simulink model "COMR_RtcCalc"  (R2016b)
settings: Solver=FixedStepDiscrete  StartTime=0.0  StopTime=10.0  FixedStep=0.1  RelTol=1e-3  EnableMultiTasking=on
undefined symbols (not defined in the file or in its folder): bin2dec, COMR_tiT37FVld_C, COMR_tiTmt2_C
libraries: simulink x3

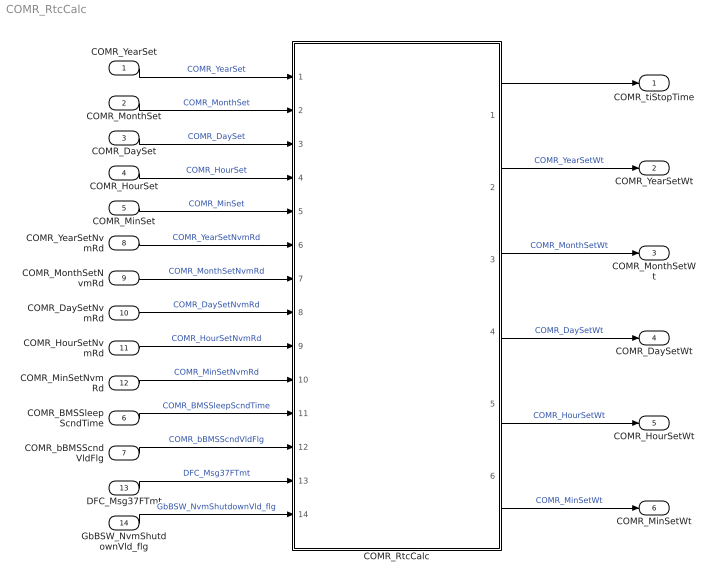
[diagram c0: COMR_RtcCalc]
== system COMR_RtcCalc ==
  COMR_YearSet : Inport
  COMR_MonthSet : Inport  Port=2
  COMR_DaySet : Inport  Port=3
  COMR_HourSet : Inport  Port=4
  COMR_MinSet : Inport  Port=5
  COMR_BMSSleepScndTime : Inport  Port=6
  COMR_bBMSScndVldFlg : Inport  Port=7
  COMR_YearSetNvmRd : Inport  Port=8
  COMR_MonthSetNvmRd : Inport  Port=9
  COMR_DaySetNvmRd : Inport  Port=10
  COMR_HourSetNvmRd : Inport  Port=11
  COMR_MinSetNvmRd : Inport  Port=12
  DFC_Msg37FTmt : Inport  Port=13
  GbBSW_NvmShutdownVld_flg : Inport  Port=14
  COMR_RtcCalc : Subsystem
  COMR_tiStopTime : Outport
  COMR_YearSetWt : Outport  Port=2  InitialOutput=[0]
  COMR_MonthSetWt : Outport  Port=3  InitialOutput=[0]
  COMR_DaySetWt : Outport  Port=4  InitialOutput=[0]
  COMR_HourSetWt : Outport  Port=5  InitialOutput=[0]
  COMR_MinSetWt : Outport  Port=6  InitialOutput=[0]
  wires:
  COMR_YearSet/1 -> COMR_RtcCalc/1(COMR_YearSet)  "COMR_YearSet"
  COMR_MonthSet/1 -> COMR_RtcCalc/2(COMR_MonthSet)  "COMR_MonthSet"
  COMR_DaySet/1 -> COMR_RtcCalc/3(COMR_DaySet)  "COMR_DaySet"
  COMR_HourSet/1 -> COMR_RtcCalc/4(COMR_HourSet)  "COMR_HourSet"
  COMR_RtcCalc/1(COMR_tiStopTime) -> COMR_tiStopTime/1
  COMR_BMSSleepScndTime/1 -> COMR_RtcCalc/11(COMR_BMSSleepScndTime)  "COMR_BMSSleepScndTime"
  COMR_bBMSScndVldFlg/1 -> COMR_RtcCalc/12(COMR_bBMSScndVldFlg)  "COMR_bBMSScndVldFlg"
  COMR_MinSet/1 -> COMR_RtcCalc/5(COMR_MinSet)  "COMR_MinSet"
  COMR_YearSetNvmRd/1 -> COMR_RtcCalc/6(COMR_YearSetNvmRd)  "COMR_YearSetNvmRd"
  COMR_MonthSetNvmRd/1 -> COMR_RtcCalc/7(COMR_MonthSetNvmRd)  "COMR_MonthSetNvmRd"
  COMR_DaySetNvmRd/1 -> COMR_RtcCalc/8(COMR_DaySetNvmRd)  "COMR_DaySetNvmRd"
  COMR_HourSetNvmRd/1 -> COMR_RtcCalc/9(COMR_HourSetNvmRd)  "COMR_HourSetNvmRd"
  COMR_MinSetNvmRd/1 -> COMR_RtcCalc/10(COMR_MinSetNvmRd)  "COMR_MinSetNvmRd"
  COMR_RtcCalc/2(COMR_YearSetWt) -> COMR_YearSetWt/1  "COMR_YearSetWt"
  COMR_RtcCalc/3(COMR_MonthSetWt) -> COMR_MonthSetWt/1  "COMR_MonthSetWt"
  COMR_RtcCalc/4(COMR_DaySetWt) -> COMR_DaySetWt/1  "COMR_DaySetWt"
  COMR_RtcCalc/5(COMR_HourSetWt) -> COMR_HourSetWt/1  "COMR_HourSetWt"
  COMR_RtcCalc/6(COMR_MinSetWt) -> COMR_MinSetWt/1  "COMR_MinSetWt"
  DFC_Msg37FTmt/1 -> COMR_RtcCalc/13(DFC_Msg37FTmt)  "DFC_Msg37FTmt"
  GbBSW_NvmShutdownVld_flg/1 -> COMR_RtcCalc/14(GbBSW_NvmShutdownVld_flg)  "GbBSW_NvmShutdownVld_flg"

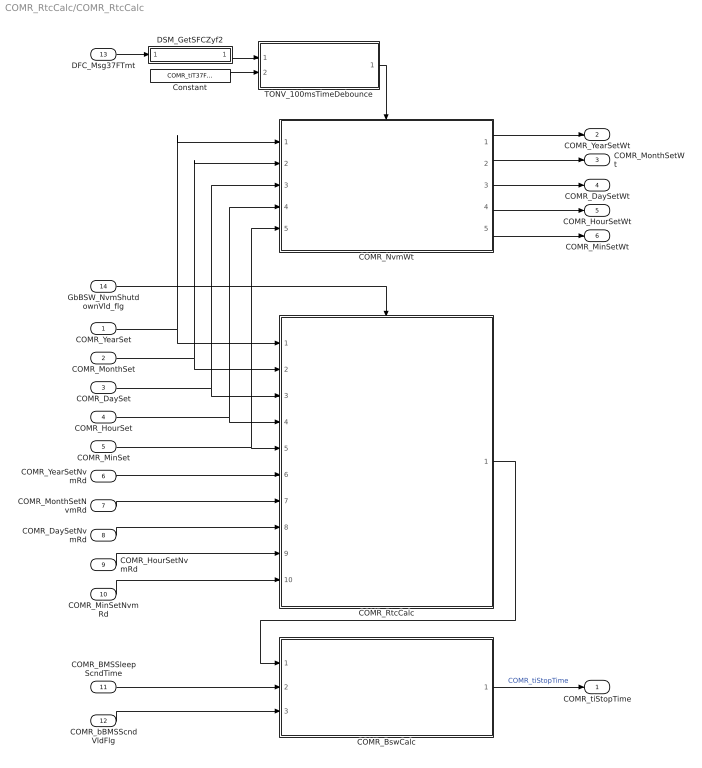
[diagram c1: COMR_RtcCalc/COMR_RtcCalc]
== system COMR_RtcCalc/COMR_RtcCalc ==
  COMR_YearSet : Inport
  COMR_MonthSet : Inport  Port=2
  COMR_DaySet : Inport  Port=3
  COMR_HourSet : Inport  Port=4
  COMR_MinSet : Inport  Port=5
  COMR_YearSetNvmRd : Inport  Port=6
  COMR_MonthSetNvmRd : Inport  Port=7
  COMR_DaySetNvmRd : Inport  Port=8
  COMR_HourSetNvmRd : Inport  Port=9
  COMR_MinSetNvmRd : Inport  Port=10
  COMR_BMSSleepScndTime : Inport  Port=11
  COMR_bBMSScndVldFlg : Inport  Port=12
  DFC_Msg37FTmt : Inport  Port=13
  GbBSW_NvmShutdownVld_flg : Inport  Port=14
  COMR_BswCalc : Subsystem
  COMR_NvmWt : Subsystem
  COMR_RtcCalc : Subsystem
  Constant : Constant  Value=COMR_tiT37FVld_C
  DSM_GetSFCZyf2 : Subsystem  TreatAsAtomicUnit=on  RTWFcnName=TONV_10msTimeDebounce  RTWFileName=SrvLib
  TONV_100msTimeDebounce : Subsystem  TreatAsAtomicUnit=on  RTWFcnName=TONV_100msTimeDebounce  RTWFileName=SrvLib
  COMR_tiStopTime : Outport
  COMR_YearSetWt : Outport  Port=2  InitialOutput=[0]
  COMR_MonthSetWt : Outport  Port=3  InitialOutput=[0]
  COMR_DaySetWt : Outport  Port=4  InitialOutput=[0]
  COMR_HourSetWt : Outport  Port=5  InitialOutput=[0]
  COMR_MinSetWt : Outport  Port=6  InitialOutput=[0]
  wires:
  COMR_YearSetNvmRd/1 -> COMR_RtcCalc/6(COMR_YearSetNvmRd)
  COMR_MonthSetNvmRd/1 -> COMR_RtcCalc/7(COMR_MonthSetNvmRd)
  COMR_MonthSet/1 -> COMR_NvmWt/2(In2), COMR_RtcCalc/2(COMR_MonthSet)
  COMR_DaySet/1 -> COMR_NvmWt/3(In3), COMR_RtcCalc/3(COMR_DaySet)
  COMR_HourSet/1 -> COMR_NvmWt/4(In4), COMR_RtcCalc/4(COMR_HourSet)
  COMR_MinSetNvmRd/1 -> COMR_RtcCalc/10(COMR_MinSetNvmRd)
  COMR_BswCalc/1(COMR_tiStopTime) -> COMR_tiStopTime/1  "COMR_tiStopTime"
  COMR_DaySetNvmRd/1 -> COMR_RtcCalc/8(COMR_DaySetNvmRd)
  COMR_HourSetNvmRd/1 -> COMR_RtcCalc/9(COMR_HourSetNvmRd)
  COMR_YearSet/1 -> COMR_NvmWt/1(In1), COMR_RtcCalc/1(COMR_YearSet)
  COMR_BMSSleepScndTime/1 -> COMR_BswCalc/2(COMR_BMSSleepScndTime)
  COMR_bBMSScndVldFlg/1 -> COMR_BswCalc/3(COMR_bBMSScndVldFlg)
  COMR_RtcCalc/1(COMR_tiStopRtcTime) -> COMR_BswCalc/1(COMR_tiStopRtcTime)
  COMR_MinSet/1 -> COMR_NvmWt/5(In5), COMR_RtcCalc/5(COMR_MinSet)
  COMR_NvmWt/1(COMR_YearSetWt) -> COMR_YearSetWt/1
  COMR_NvmWt/2(COMR_MonthSetWt) -> COMR_MonthSetWt/1
  COMR_NvmWt/3(COMR_DaySetWt) -> COMR_DaySetWt/1
  COMR_NvmWt/4(COMR_HourSetWt) -> COMR_HourSetWt/1
  COMR_NvmWt/5(COMR_MinSetWt) -> COMR_MinSetWt/1
  Constant/1 -> TONV_100msTimeDebounce/2(T)
  TONV_100msTimeDebounce/1(y) -> COMR_NvmWt/Enable
  DSM_GetSFCZyf2/1(y) -> TONV_100msTimeDebounce/1(u)
  DFC_Msg37FTmt/1 -> DSM_GetSFCZyf2/1(DFC)
  GbBSW_NvmShutdownVld_flg/1 -> COMR_RtcCalc/Enable

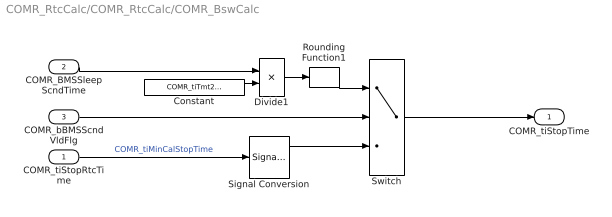
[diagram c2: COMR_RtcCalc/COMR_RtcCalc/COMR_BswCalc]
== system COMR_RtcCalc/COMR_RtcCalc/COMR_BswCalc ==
  COMR_tiStopRtcTime : Inport
  COMR_BMSSleepScndTime : Inport  Port=2
  COMR_bBMSScndVldFlg : Inport  Port=3
  Constant : Constant  Value=COMR_tiTmt2_C  OutDataTypeStr=single
  Divide1 : Product  Inputs=*/
  Rounding Function1 : Rounding
  Signal Conversion : SignalConversion  OverrideOpt=off
  Switch : Switch  Criteria=u2 ~= 0
  COMR_tiStopTime : Outport
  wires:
  COMR_bBMSScndVldFlg/1 -> Switch/2
  COMR_BMSSleepScndTime/1 -> Divide1/1
  COMR_tiStopRtcTime/1 -> Signal Conversion/1  "COMR_tiMinCalStopTime"
  Switch/1 -> COMR_tiStopTime/1
  Rounding Function1/1 -> Switch/1
  Constant/1 -> Divide1/2
  Divide1/1 -> Rounding Function1/1
  Signal Conversion/1 -> Switch/3

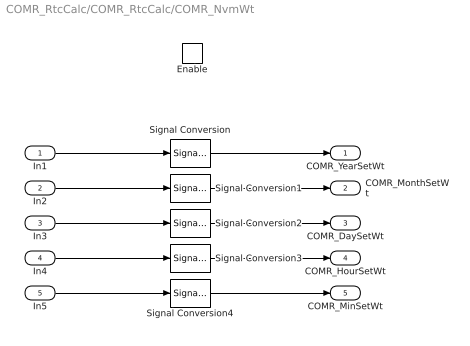
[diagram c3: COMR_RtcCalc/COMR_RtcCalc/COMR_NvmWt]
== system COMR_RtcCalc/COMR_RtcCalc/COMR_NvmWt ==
  In1 : Inport
  In2 : Inport  Port=2
  In3 : Inport  Port=3
  In4 : Inport  Port=4
  In5 : Inport  Port=5
  Enable : EnablePort  StatesWhenEnabling=reset
  Signal Conversion{,1..4} (5 alike) : SignalConversion  OverrideOpt=off
  COMR_YearSetWt : Outport  InitialOutput=[0]
  COMR_MonthSetWt : Outport  Port=2  InitialOutput=[0]
  COMR_DaySetWt : Outport  Port=3  InitialOutput=[0]
  COMR_HourSetWt : Outport  Port=4  InitialOutput=[0]
  COMR_MinSetWt : Outport  Port=5  InitialOutput=[0]
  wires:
  In3/1 -> Signal Conversion2/1
  Signal Conversion/1 -> COMR_YearSetWt/1
  Signal Conversion1/1 -> COMR_MonthSetWt/1
  In1/1 -> Signal Conversion/1
  Signal Conversion2/1 -> COMR_DaySetWt/1
  Signal Conversion3/1 -> COMR_HourSetWt/1
  Signal Conversion4/1 -> COMR_MinSetWt/1
  In4/1 -> Signal Conversion3/1
  In2/1 -> Signal Conversion1/1
  In5/1 -> Signal Conversion4/1

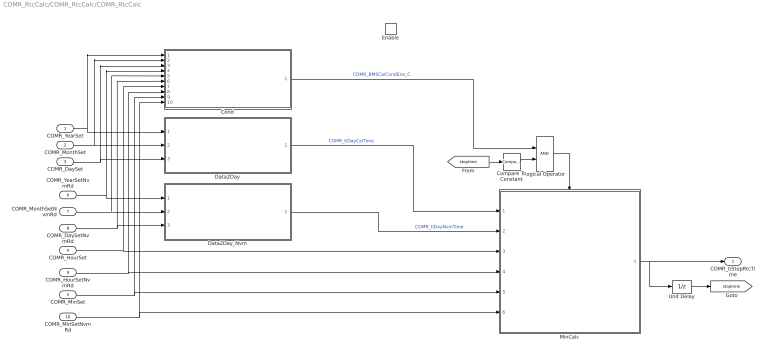
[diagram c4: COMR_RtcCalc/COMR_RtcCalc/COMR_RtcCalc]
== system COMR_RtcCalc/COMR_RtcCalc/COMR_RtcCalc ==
  COMR_YearSet : Inport
  COMR_MonthSet : Inport  Port=2
  COMR_DaySet : Inport  Port=3
  COMR_HourSet : Inport  Port=4
  COMR_MinSet : Inport  Port=5
  COMR_YearSetNvmRd : Inport  Port=6
  COMR_MonthSetNvmRd : Inport  Port=7
  COMR_DaySetNvmRd : Inport  Port=8
  COMR_HourSetNvmRd : Inport  Port=9
  COMR_MinSetNvmRd : Inport  Port=10
  Enable : EnablePort  StatesWhenEnabling=reset
  Compare To Constant : simulink/Logic and Bit Operations/Compare To Constant  relop=<=  const=0  OutDataTypeStr=boolean
  Cond : Subsystem
  Data2Day : Subsystem
  Data2Day_Nvm : Subsystem
  Logical Operator : Logic  AllPortsSameDT=off  OutDataTypeStr=boolean
  MinCalc : Subsystem
  Unit Delay : UnitDelay  SampleTime=-1
  COMR_tiStopRtcTime : Outport  InitialOutput=[0]
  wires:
  MinCalc/1(COMR_tiStopTime) -> Unit Delay/1, COMR_tiStopRtcTime/1
  COMR_YearSet/1 -> Cond/1(COMR_BMSYear), Data2Day/1(BSER_tiYearSet)
  COMR_DaySet/1 -> Cond/3(COMR_BMSDay), Data2Day/3(BSER_tiDaySet)
  COMR_MonthSet/1 -> Cond/2(COMR_BMSMonth), Data2Day/2(BSER_tiMonthSet)
  COMR_YearSetNvmRd/1 -> Cond/4(COMR_BMSYear_nvm), Data2Day_Nvm/1(COMR_BMSYear_nvm)
  COMR_MonthSetNvmRd/1 -> Cond/5(COMR_BMSMonth_nvm), Data2Day_Nvm/2(COMR_BMSMonth_nvm)
  COMR_DaySetNvmRd/1 -> Cond/6(COMR_BMSDay_nvm), Data2Day_Nvm/3(COMR_BMSDay_nvm)
  COMR_HourSet/1 -> Cond/7(COMR_BMSHour), MinCalc/3(COMR_BMSHour)
  COMR_HourSetNvmRd/1 -> Cond/8(COMR_BMSHour_nvm), MinCalc/4(COMR_BMSHour_nvm)
  COMR_MinSetNvmRd/1 -> Cond/10(COMR_BMSMinute_nvm), MinCalc/6(COMR_BMSMinute_nvm)
  COMR_MinSet/1 -> Cond/9(COMR_BMSMinute), MinCalc/5(COMR_BMSMinute)
  Data2Day/1(BSER_tiDay) -> MinCalc/1(BSER_tiDay)  "COMR_tiDayCalTime"
  Data2Day_Nvm/1(BSER_tiDay_nvm) -> MinCalc/2(BSER_tiDay_nvm)  "COMR_tiDayNvmTime"
  Cond/1(COMR_bStopTimeCalcEn) -> Logical Operator/1  "COMR_BMSCalCondEna_C"
  Compare To Constant/1 -> Logical Operator/2
  [stoptime] -> Compare To Constant/1
  Logical Operator/1 -> MinCalc/Enable
  Unit Delay/1 -> [stoptime]

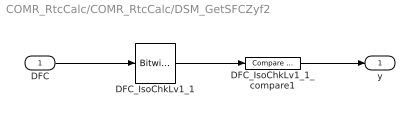
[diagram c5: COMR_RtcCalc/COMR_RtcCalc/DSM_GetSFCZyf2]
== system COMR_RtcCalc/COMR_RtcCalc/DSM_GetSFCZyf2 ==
  DFC : Inport  OutDataTypeStr=uint8
  DFC_IsoChkLv1_1 : simulink/Logic and Bit Operations/Bitwise Operator  logicop=AND  UseBitMask=on  BitMask=bin2dec('00001000')  BitMaskRealWorld=Stored Integer
  DFC_IsoChkLv1_1_compare1 : simulink/Logic and Bit Operations/Compare To Constant  relop===  const=8  OutDataTypeStr=boolean
  y : Outport
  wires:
  DFC_IsoChkLv1_1/1 -> DFC_IsoChkLv1_1_compare1/1
  DFC/1 -> DFC_IsoChkLv1_1/1
  DFC_IsoChkLv1_1_compare1/1 -> y/1

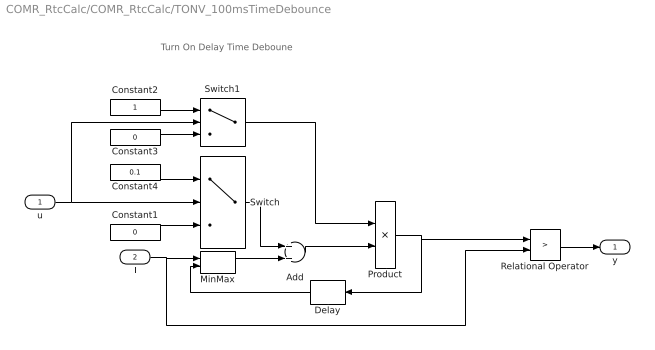
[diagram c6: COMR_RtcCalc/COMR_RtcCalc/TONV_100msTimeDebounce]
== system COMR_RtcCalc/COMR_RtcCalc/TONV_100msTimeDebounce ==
  note: Turn On Delay Time Deboune
  u : Inport
  T : Inport  Port=2
  Add : Sum
  Constant1 : Constant  Value=0  OutDataTypeStr=single
  Constant2 : Constant  OutDataTypeStr=uint8
  Constant3 : Constant  Value=0  OutDataTypeStr=uint8
  Constant4 : Constant  Value=0.1  OutDataTypeStr=single
  Delay : Delay  DelayLength=1  InitialCondition=0
  MinMax : MinMax  Inputs=2
  Product : Product  OutMin=[0]  OutMax=[65535]  OutDataTypeStr=single
  Relational Operator : RelationalOperator  Operator=>  OutDataTypeStr=boolean  RndMeth=Simplest
  Switch : Switch  Criteria=u2 ~= 0
  Switch1 : Switch  Criteria=u2 ~= 0
  y : Outport
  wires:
  Switch1/1 -> Product/1
  Constant3/1 -> Switch1/3
  Constant2/1 -> Switch1/1
  u/1 -> Switch1/2, Switch/2
  Constant4/1 -> Switch/1
  Constant1/1 -> Switch/3
  Add/1 -> Product/2
  Product/1 -> Relational Operator/1, Delay/1
  Switch/1 -> Add/1
  Delay/1 -> MinMax/2
  Relational Operator/1 -> y/1
  T/1 -> MinMax/1, Relational Operator/2
  MinMax/1 -> Add/2

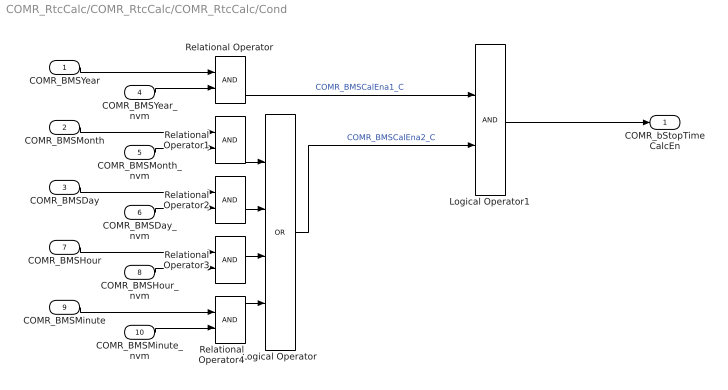
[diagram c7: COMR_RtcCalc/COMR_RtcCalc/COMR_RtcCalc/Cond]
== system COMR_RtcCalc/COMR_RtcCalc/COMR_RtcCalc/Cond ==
  COMR_BMSYear : Inport
  COMR_BMSMonth : Inport  Port=2
  COMR_BMSDay : Inport  Port=3
  COMR_BMSYear_nvm : Inport  Port=4
  COMR_BMSMonth_nvm : Inport  Port=5
  COMR_BMSDay_nvm : Inport  Port=6
  COMR_BMSHour : Inport  Port=7
  COMR_BMSHour_nvm : Inport  Port=8
  COMR_BMSMinute : Inport  Port=9
  COMR_BMSMinute_nvm : Inport  Port=10
  Logical Operator : Logic  Operator=OR  Inputs=4  AllPortsSameDT=off  OutDataTypeStr=boolean
  Logical Operator1 : Logic  AllPortsSameDT=off  OutDataTypeStr=boolean
  Relational Operator{,1..4} (5 alike) : RelationalOperator  OutDataTypeStr=boolean  RndMeth=Simplest
  COMR_bStopTimeCalcEn : Outport
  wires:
  COMR_BMSYear/1 -> Relational Operator/1
  COMR_BMSYear_nvm/1 -> Relational Operator/2
  COMR_BMSMonth/1 -> Relational Operator1/1
  COMR_BMSMonth_nvm/1 -> Relational Operator1/2
  COMR_BMSDay/1 -> Relational Operator2/1
  COMR_BMSDay_nvm/1 -> Relational Operator2/2
  COMR_BMSHour/1 -> Relational Operator3/1
  COMR_BMSHour_nvm/1 -> Relational Operator3/2
  COMR_BMSMinute/1 -> Relational Operator4/1
  COMR_BMSMinute_nvm/1 -> Relational Operator4/2
  Relational Operator1/1 -> Logical Operator/1
  Relational Operator2/1 -> Logical Operator/2
  Relational Operator3/1 -> Logical Operator/3
  Relational Operator4/1 -> Logical Operator/4
  Logical Operator/1 -> Logical Operator1/2  "COMR_BMSCalEna2_C"
  Relational Operator/1 -> Logical Operator1/1  "COMR_BMSCalEna1_C"
  Logical Operator1/1 -> COMR_bStopTimeCalcEn/1

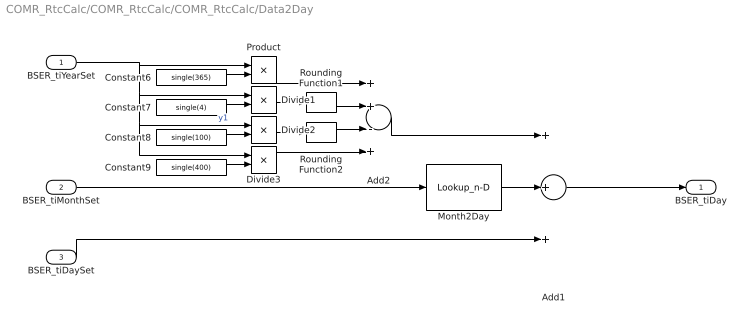
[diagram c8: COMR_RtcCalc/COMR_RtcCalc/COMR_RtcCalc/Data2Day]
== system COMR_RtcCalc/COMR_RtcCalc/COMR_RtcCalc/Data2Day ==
  BSER_tiYearSet : Inport
  BSER_tiMonthSet : Inport  Port=2
  BSER_tiDaySet : Inport  Port=3
  Add1 : Sum  Inputs=+++
  Add2 : Sum  Inputs=++-+
  Constant6 : Constant  Value=single(365)
  Constant7 : Constant  Value=single(4)
  Constant8 : Constant  Value=single(100)
  Constant9 : Constant  Value=single(400)
  Divide1 : Product  Inputs=*/
  Divide2 : Product  Inputs=*/
  Divide3 : Product  Inputs=*/
  Month2Day : Lookup_n-D  NumberOfTableDimensions=1  BreakpointsForDimension1=[1 2 3 4 5 6 7 8 9 10 11 12]  Table=[0 31 59 90 120 151 181 212 243 273 304 334]  InterpMethod=Flat  InternalRulePriority=Speed  OutDataTypeStr=single  RndMeth=Simplest
  Product : Product
  Rounding Function1 : Rounding
  Rounding Function2 : Rounding
  BSER_tiDay : Outport
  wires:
  Constant8/1 -> Divide2/2
  Divide2/1 -> Rounding Function2/1
  Add1/1 -> BSER_tiDay/1
  BSER_tiYearSet/1 -> Divide2/1, Divide3/1, Divide1/1, Product/1  "y1"
  BSER_tiMonthSet/1 -> Month2Day/1
  Constant6/1 -> Product/2
  Divide1/1 -> Rounding Function1/1
  Month2Day/1 -> Add1/2
  Constant7/1 -> Divide1/2
  Constant9/1 -> Divide3/2
  Product/1 -> Add2/1
  Rounding Function1/1 -> Add2/2
  Rounding Function2/1 -> Add2/3
  Divide3/1 -> Add2/4
  Add2/1 -> Add1/1
  BSER_tiDaySet/1 -> Add1/3

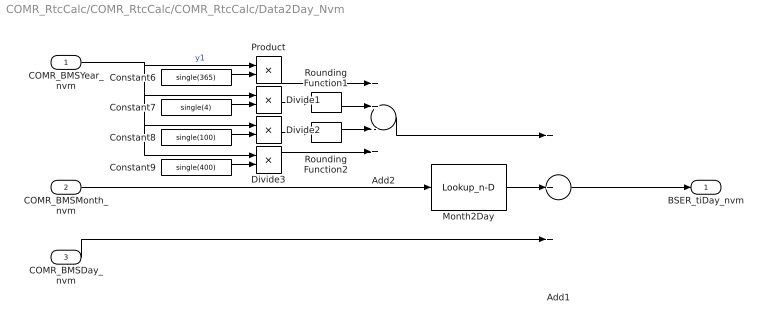
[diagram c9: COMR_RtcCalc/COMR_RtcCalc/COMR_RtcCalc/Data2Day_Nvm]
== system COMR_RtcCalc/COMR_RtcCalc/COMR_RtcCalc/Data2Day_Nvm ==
  COMR_BMSYear_nvm : Inport
  COMR_BMSMonth_nvm : Inport  Port=2
  COMR_BMSDay_nvm : Inport  Port=3
  Add1 : Sum  Inputs=+++
  Add2 : Sum  Inputs=++-+
  Constant6 : Constant  Value=single(365)
  Constant7 : Constant  Value=single(4)
  Constant8 : Constant  Value=single(100)
  Constant9 : Constant  Value=single(400)
  Divide1 : Product  Inputs=*/
  Divide2 : Product  Inputs=*/
  Divide3 : Product  Inputs=*/
  Month2Day : Lookup_n-D  NumberOfTableDimensions=1  BreakpointsForDimension1=[1 2 3 4 5 6 7 8 9 10 11 12]  Table=[0 31 59 90 120 151 181 212 243 273 304 334]  InterpMethod=Flat  InternalRulePriority=Speed  OutDataTypeStr=single  RndMeth=Simplest
  Product : Product
  Rounding Function1 : Rounding
  Rounding Function2 : Rounding
  BSER_tiDay_nvm : Outport
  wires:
  Add2/1 -> Add1/1
  Divide3/1 -> Add2/4
  Rounding Function2/1 -> Add2/3
  Rounding Function1/1 -> Add2/2
  Product/1 -> Add2/1
  Constant9/1 -> Divide3/2
  Constant7/1 -> Divide1/2
  Month2Day/1 -> Add1/2
  Divide1/1 -> Rounding Function1/1
  Constant6/1 -> Product/2
  COMR_BMSMonth_nvm/1 -> Month2Day/1
  COMR_BMSYear_nvm/1 -> Product/1, Divide1/1, Divide3/1, Divide2/1  "y1"
  Add1/1 -> BSER_tiDay_nvm/1
  Divide2/1 -> Rounding Function2/1
  Constant8/1 -> Divide2/2
  COMR_BMSDay_nvm/1 -> Add1/3

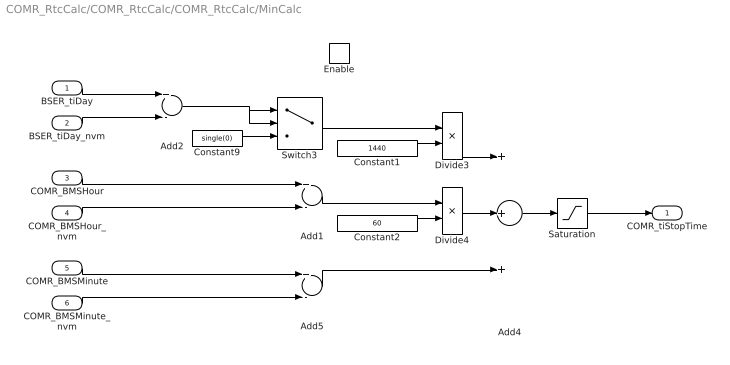
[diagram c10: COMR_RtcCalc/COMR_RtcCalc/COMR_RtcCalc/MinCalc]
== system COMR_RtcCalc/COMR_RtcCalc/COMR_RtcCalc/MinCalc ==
  BSER_tiDay : Inport
  BSER_tiDay_nvm : Inport  Port=2
  COMR_BMSHour : Inport  Port=3
  COMR_BMSHour_nvm : Inport  Port=4
  COMR_BMSMinute : Inport  Port=5
  COMR_BMSMinute_nvm : Inport  Port=6
  Enable : EnablePort  StatesWhenEnabling=reset
  Add1 : Sum  Inputs=+-  OutDataTypeStr=int16
  Add2 : Sum  Inputs=+-  OutDataTypeStr=int16
  Add4 : Sum  Inputs=+++
  Add5 : Sum  Inputs=+-  OutDataTypeStr=int16
  Constant1 : Constant  Value=1440  OutDataTypeStr=uint16
  Constant2 : Constant  Value=60  OutDataTypeStr=uint16
  Constant9 : Constant  Value=single(0)  OutDataTypeStr=uint8
  Divide3 : Product  Inputs=**  OutDataTypeStr=single
  Divide4 : Product  Inputs=**  OutDataTypeStr=single
  Saturation : Saturate  UpperLimit=1000000000  LowerLimit=0
  Switch3 : Switch
  COMR_tiStopTime : Outport
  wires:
  COMR_BMSHour/1 -> Add1/1
  COMR_BMSHour_nvm/1 -> Add1/2
  Constant1/1 -> Divide3/2
  Add4/1 -> Saturation/1
  Add2/1 -> Switch3/2, Switch3/1
  Constant9/1 -> Switch3/3
  BSER_tiDay/1 -> Add2/1
  BSER_tiDay_nvm/1 -> Add2/2
  COMR_BMSMinute/1 -> Add5/1
  COMR_BMSMinute_nvm/1 -> Add5/2
  Switch3/1 -> Divide3/1
  Constant2/1 -> Divide4/2
  Add1/1 -> Divide4/1
  Divide3/1 -> Add4/1
  Divide4/1 -> Add4/2
  Add5/1 -> Add4/3
  Saturation/1 -> COMR_tiStopTime/1
